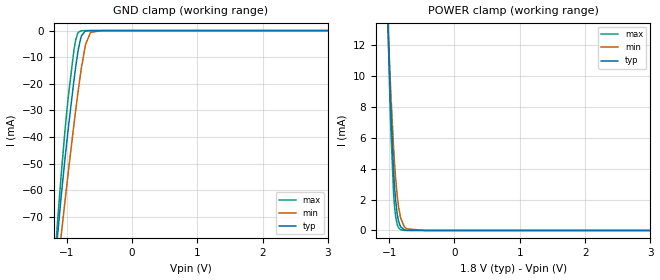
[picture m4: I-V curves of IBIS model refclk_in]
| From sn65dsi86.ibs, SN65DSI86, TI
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|   Model
[Model]   refclk_in
Model_type   Input
Vinl = 0.54
Vinh = 1.26
|   typ   min   max
C_comp   1.198pF   1.124pF   1.275pF
[Voltage Range]   1.8   1.65   1.98
[Temperature Range]   27   125   -40
[Power Clamp Reference]   1.8   1.65   1.98
[GND Clamp Reference]   -0   -0   -0
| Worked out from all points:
|   GND clamp passes 1 mA (typ) near -0.74 V on its own axis
|   POWER clamp passes 1 mA (typ) near -0.87 V on its own axis
[GND Clamp]
|   Voltage   I(typ)   I(min)   I(max)
-1.8V     -308mA     -294.7mA   -317.4mA
-1.217V   -100.4mA   -108.4mA   -98.82mA
-1.141V   -77.87mA   -90.3mA    -72.89mA
-1.087V   -63.42mA   -77.98mA   -55.59mA
-1.028V   -48.94mA   -64.84mA   -38.42mA
-968.4mV  -35.52mA   -52.05mA   -23.65mA
-887.4mV  -18.7mA    -35.25mA   -7.366mA
-817.2mV  -6.639mA   -21.68mA   -578.5uA
-774mV    -2.027mA   -14.15mA   -80.7uA
-714.6mV  -173.1uA   -5.777mA   -5.698uA
-633.6mV  -4.37uA    -642.7uA   -124.7nA
3.595V    0A         0A         0A
[POWER Clamp]
|   Voltage   I(typ)   I(min)   I(max)
-1.8V     160.5mA    133.1mA    189mA
-1.028V   14.8mA     14.6mA     14.8mA
-984.6mV  9.086mA    9.953mA    8.012mA
-973.8mV  7.836mA    8.907mA    6.583mA
-930.6mV  3.782mA    5.297mA    2.365mA
-903.6mV  2.114mA    3.571mA    1.016mA
-876.6mV  1.079mA    2.275mA    388.8uA
-828mV    275.3uA    892.3uA    60.77uA
-768.6mV  46.49uA    247.8uA    5.945uA
-730.8mV  14.74uA    105.8uA    1.344uA
-450mV    0A         160.6nA    0A
3.595V    0A         0A         0A
